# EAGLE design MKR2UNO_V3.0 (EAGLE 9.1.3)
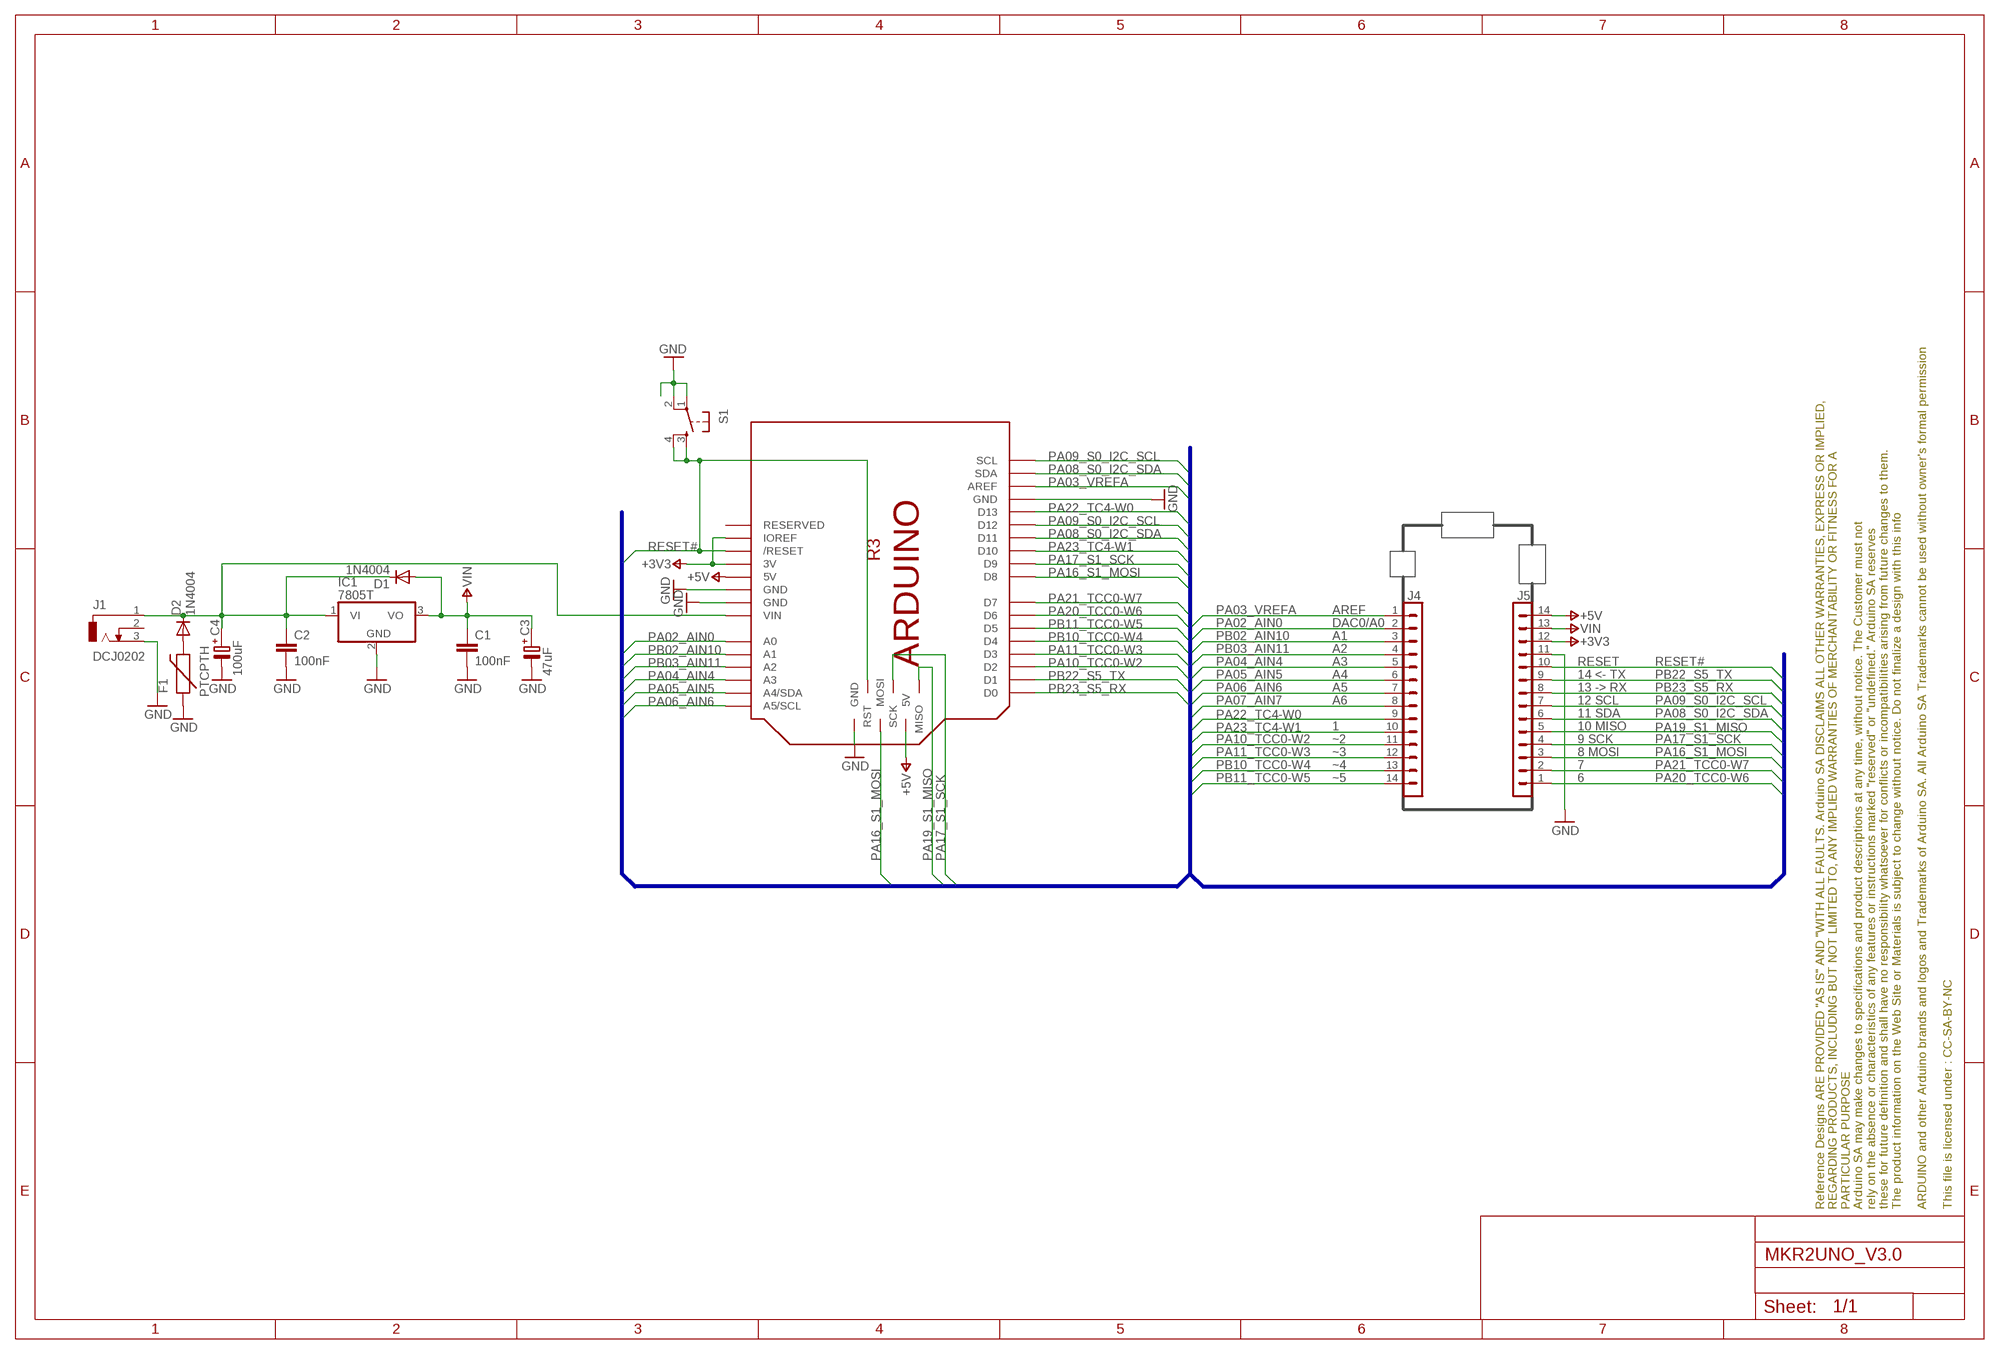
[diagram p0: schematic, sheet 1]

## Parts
C1  100nF  C-EU025-024X044  [C025-024X044]
C2  100nF  C-EU025-024X044  [C025-024X044]
C3  47uF  C-PA-6,3X10  [EA6,3-10]
C4  100uF  C-PA-6,3X10  [EA6,3-10]
D1  1N4004  [DO41-10]
D2  1N4004  [DO41-10]
F1  PTCPTH  [PTC]
FRAME1  DNP  A3-FRAME-STANDARD  [FRAME]
IC1  7805T  [TO220H]
J1  DCJ0202  [DCJ0202]
J4  DNP  STRIP-14STD  [1X14]
J5  DNP  STRIP-14STD  [1X14]
M1  ARDUINO_R3_ICSP  [ARDUINOR3_ICSP]
S1  TAC_SWITCHPTH  [TACTILE-PTH]

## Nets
+3V3: J5.12 M1.3V M1.IOREF
+5V: J5.14 M1.5V M1.5V_ICSP(5V)
GND: C1.2 C2.2 C3.- C4.- F1.P$1 IC1.2(GND) J1.3 J5.11 M1.GND M1.GND@1(GND) M1.GND@2(GND) M1.GND@3(GND) S1.1 S1.2
N$1: C2.1 C4.+ D1.C D2.C IC1.1(VI) J1.1 M1.VIN
N$2: D2.A F1.P$2
PA02_AIN0: J4.2 M1.A0
PA03_VREFA: J4.1 M1.AREF
PA04_AIN4: J4.5 M1.A3
PA05_AIN5: J4.6 M1.A4(A4/SDA)
PA06_AIN6: J4.7 M1.A5(A5/SCL)
PA07_AIN7: J4.8
PA08_S0_I2C_SDA: J5.6 M1.D11 M1.SDA
PA09_S0_I2C_SCL: J5.7 M1.D12 M1.SCL
PA10_TCC0-W2: J4.11 M1.D2
PA11_TCC0-W3: J4.12 M1.D3
PA16_S1_MOSI: J5.3 M1.D8 M1.MOSI
PA17_S1_SCK: J5.4 M1.D9 M1.SCK
PA19_S1_MISO: J5.5 M1.MISO
PA20_TCC0-W6: J5.1 M1.D6
PA21_TCC0-W7: J5.2 M1.D7
PA22_TC4-W0: J4.9 M1.D13
PA23_TC4-W1: J4.10 M1.D10
PB02_AIN10: J4.3 M1.A1
PB03_AIN11: J4.4 M1.A2
PB10_TCC0-W4: J4.13 M1.D4
PB11_TCC0-W5: J4.14 M1.D5
PB22_S5_TX: J5.9 M1.D1
PB23_S5_RX: J5.8 M1.D0
RESET#: J5.10 M1.RESET(/RESET) M1.RESET_ICSP(RST) S1.3 S1.4
VIN: C1.1 C3.+ D1.A IC1.3(VO) J5.13
Unconnected: J1.2 M1.RESERVED

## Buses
PA03_VREFA,PA02_AIN0,PB02_AIN10,PB03_AIN11PA04_AIN4,PA05_AIN5,PA06_AIN6,PA07_AIN7,PA22_TC4-W0,PA23_TC4-W1,PA10_TCC0-W2,PA11_TCC0-W3,PB10_TCC0-W4,PB11_TCC0-W5,PA20_TCC0-W6,PA21_TCC0-W7,PA16_S1_MOSI,PA17_S1_SCK,PA19_S1_MISO,PA08_S0_I2C_SDA,PA09_S0_I2C_SCL,PB23_S5_RX,PB22_S5_TX,RESET#

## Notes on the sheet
- AREF
- DAC0/A0
- A1
- A2
- A3 | RESET
- A4 | 14 <- TX
- A5 | 13 -> RX
- A6 | 12 SCL
- 11 SDA
- 1 | 10 MISO
- ~2 | 9 SCK
- ~3 | 8 MOSI
- ~4 | 7
- ~5 | 6

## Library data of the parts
C1 C2 = rcl:C-EU: CAPACITOR, European symbol
C3 C4 = cap-pan40:C-PA: POLARIZED AXIAL ELECTROLYTIC
D1 D2 = diode:1N4004: DIODE
F1 = SparkFun:PTC: Resettable Fuse PTC
FRAME1 = Arduino-utility:A3-FRAME: Schematic frame; CODE-ARDUINO: DNP; DATASHEET: DNP; DISTRIBUTOR-LINK: DNP; DISTRIBUTOR-PN: DNP; MANUFACTURER: DNP; MANUFACTURER-PN: DNP
IC1 = linear:78*: Positive VOLTAGE REGULATOR Source: http://cache.national.com/ds/LM/LM78L05.pdf http://www.fairchildsemi.com/ds/LM/LM7805.pdf
J1 = con-jack:DCJ0202: DC POWER JACK Source: DCJ0202.pdf
J4 J5 = Arduino-connectors:STRIP-14
M1 = Arduino-BoardFootprints:ARDUINO_R3_ICSP
S1 = SparkFun:TAC_SWITCH: Momentary Switch Button commonly used for reset or general input. Spark Fun Electronics SKU : COM-00097

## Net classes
0 default: width 0.25 mm, drill 0.25 mm

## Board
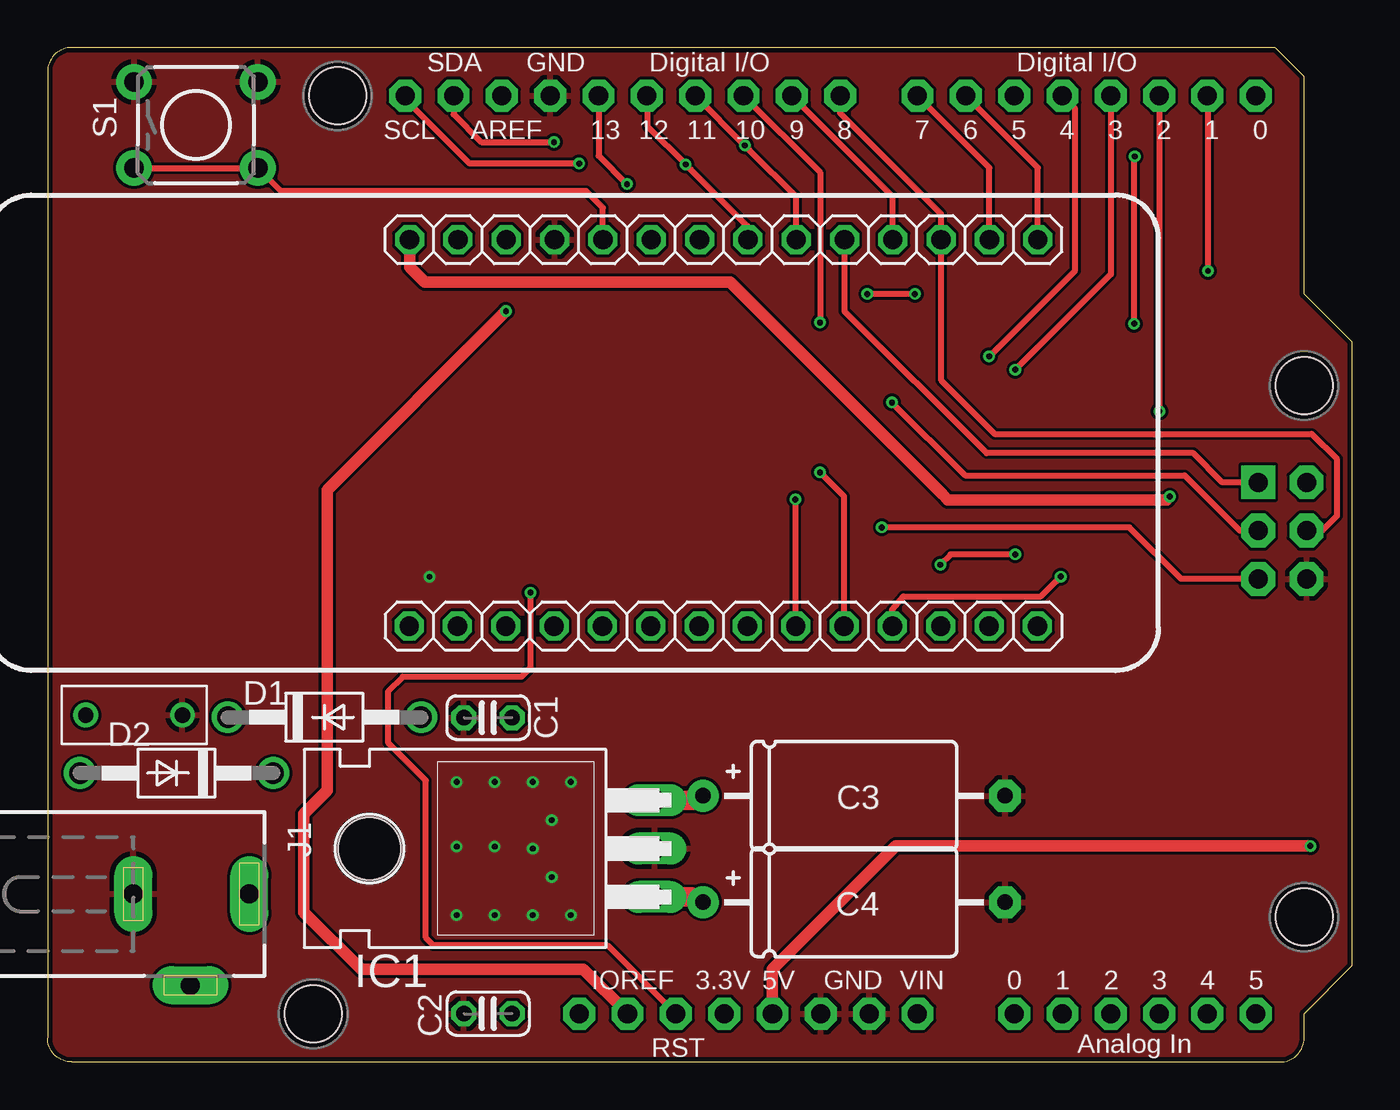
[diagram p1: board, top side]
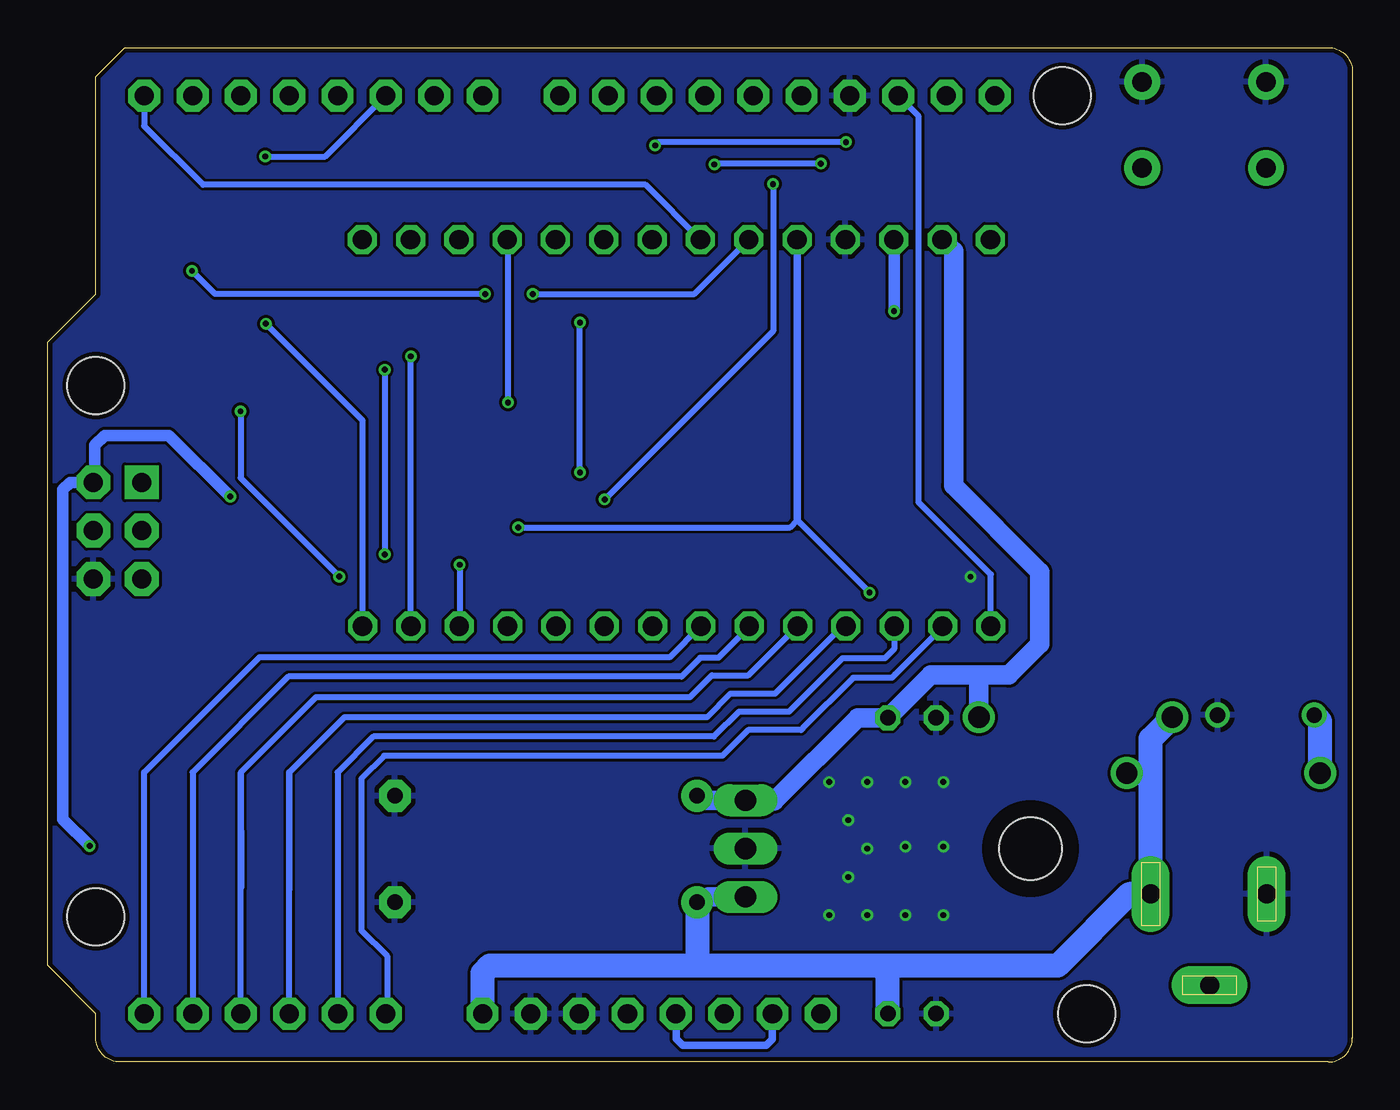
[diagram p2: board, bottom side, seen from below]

Size 68.58 x 53.34 mm. Coordinates in mm from the lower left corner, seen from the top.
Copper layers (1*16): Top 0.035mm / dielectric 1.5mm / Bottom 0.035mm
Design rules "SeeedStudio_2layers *": minimum track width 6mil, minimum drill 12mil, track to track 6mil, track to pad 6mil, pad to pad 6mil, via to via 6mil, smd to smd 0mil, copper to edge 10mil, drill to drill 10mil, minimum pad ring 10mil, minimum via ring 6mil, stop-mask expansion 2mil, vias tented up to drill 100mil, thermal gap 10mil

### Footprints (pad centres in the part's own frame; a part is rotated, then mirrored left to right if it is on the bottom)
C025-024X044 = drill 0.813 octagon: 1 -1.27,0; 2 1.27,0
EA6,3-10 = drill 0.813 pad 1.676: + -8.255,0 | drill 0.813 pad 1.676 octagon: - 7.62,0
DO41-10 = drill 1.118: A 5.08,0; C -5.08,0
PTC = drill 0.8: P$1 -2.54,0; P$2 2.54,0
TO220H = drill 1.118 long: 1 -2.54,-10.16; 2 0,-10.16; 3 2.54,-10.16 | hole 3.302: 0,4.826
DCJ0202 = drill 1 pad 2 long: 1 0,3.1; 2 4.8,0; 3 0,-3
1X14 = drill 1.016 octagon: 1 -16.51,0; 2 -13.97,0; 3 -11.43,0; 4 -8.89,0; 5 -6.35,0; 6 -3.81,0; 7 -1.27,0; 8 1.27,0; 9 3.81,0; 10 6.35,0; 11 8.89,0; 12 11.43,0; 13 13.97,0; 14 16.51,0
ARDUINOR3_ICSP = drill 1 pad 1.676 octagon: 3V 35.56,2.54; 5V 38.1,2.54; A0 50.8,2.54; A1 53.34,2.54; A2 55.88,2.54; A3 58.42,2.54; A4 60.96,2.54; A5 63.5,2.54; AREF 23.876,50.8; D0 63.5,50.8; D1 60.96,50.8; D2 58.42,50.8; D3 55.88,50.8; D4 53.34,50.8; D5 50.8,50.8; D6 48.26,50.8; D7 45.72,50.8; D8 41.656,50.8; D9 39.116,50.8; D10 36.576,50.8; D11 34.036,50.8; D12 31.496,50.8; D13 28.956,50.8; GND 26.416,50.8; GND@1 43.18,2.54; GND@2 40.64,2.54; IOREF 30.48,2.54; RESERVED 27.94,2.54; RESET 33.02,2.54; SCL 18.796,50.8; SDA 21.336,50.8; VIN 45.72,2.54 | drill 1 pad 1.778 octagon: 5V_ICSP 66.167,30.48; GND@3 66.167,25.4; MOSI 66.167,27.94; RESET_ICSP 63.627,25.4; SCK 63.627,27.94 | drill 1 pad 1.778 square: MISO 63.627,30.48 | hole 3: 15.24,50.8; 13.97,2.54; 66.04,7.62; 66.04,35.56
TACTILE-PTH = drill 1.016 pad 1.88: 1 -3.251,2.261; 2 3.251,2.261; 3 -3.251,-2.261; 4 3.251,-2.261

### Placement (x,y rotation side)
C1  23.15,18.1 180 top
C2  23.15,2.54 180 top
C3  42.7,14 0 top
C4  42.7,8.4 0 top
D1  14.55,18.13 0 top
D2  6.78,15.19 180 top
F1  4.55,18.24 180 top
FRAME1  not placed on the board
IC1  21.74,11.22 90 top
J1  7.51,8.83 270 top
J4  35.51,22.92 0 top
J5  35.53,43.24 180 top
M1  0,0 0 top
S1  7.8,49.27 0 top

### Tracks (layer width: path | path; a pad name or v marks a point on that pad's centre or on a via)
+3V3  (via drill 0.3 pad 0.61)
  Top 0.61: M1.IOREF 28.16,4.87 16.48,4.87 13.47,7.88 13.47,13.05 14.69,14.27 14.69,30.08 v24.09,39.48 24.07,39.5
  Bottom 0.406: M1.IOREF 30.48,1.19 30.8,0.87 35.19,0.87 35.54,1.22 35.54,2.52 M1.3V
  Bottom 0.61: v24.09,39.48 24.09,43.23 J5.12
+5V  (via drill 0.3, 0.3 pad 0.61)
  Top 0.61: v58.98,29.73 58.81,29.56 47.31,29.56 47.04,29.83 47.04,29.84 35.87,41.01 19.82,41.01 19.02,41.8 J5.14 | v66.37,11.36 46.92,11.36 46.91,11.37 44.59,11.37 38.1,4.88 M1.5V
  Bottom 0.61: v58.98,29.73 62.2,32.95 65.58,32.95 66.1,32.43 66.1,30.55 M1.5V_ICSP 67.4,30.48 67.77,30.11 67.77,12.76 v66.37,11.36
GND  (via drill 0.3)
  other vias: 27.5,7.72 25.5,7.72 23.5,7.72 21.5,7.72 27.5,14.72 26.5,12.72 26.5,9.72 25.5,11.22 23.5,11.32 21.5,11.32 25.5,14.72 23.5,14.72 21.5,14.72 20.07,25.51
  pour Bottom: 0,55 70,55 70,0 0,0
  pour Top: 0,55 70,55 70,0 0,0
N$1
  Top 1.016: IC1.1 33.84,8.68 C4.+
  Bottom 0.406: 16.69,5.07 16.74,5.07 16.74,5.4
  Bottom 1.016: 34.12,5.13 34.05,5.07 | C4.+ 33.84,8.68 31.82,8.68
  Bottom 1.27: M1.VIN 45.72,4.67 45.32,5.07 34.05,5.07 24.85,5.07 | 24.85,5.07 16.69,5.07 16.68,5.06 15.5,5.06 11.73,8.83 J1.1 10.61,14.94 | C2.1 24.42,4.64 24.85,5.07 | 10.61,14.94 10.61,16.99 D1.C | C4.+ 34.45,5.46 34.12,5.13 | D2.C 10.86,15.19 10.61,14.94
N$2
  Bottom 1.27: D2.A 1.7,17.93 F1.P$2
PA02_AIN0
  Bottom 0.305: J4.2 21.55,22.88 24.03,20.39 24.03,20.38 24.21,20.2 26.24,20.2 28.88,17.56 28.88,17.55 28.98,17.45 31.76,17.45 33.11,16.1 50.89,16.1 52.09,14.9 52.09,6.92 50.74,5.57 50.74,2.6 M1.A0
PA03_VREFA
  Bottom 0.305: M1.AREF 22.8,49.72 22.8,29.43 19,25.64 J4.1
PA04_AIN4
  Bottom 0.305: 58.49,2.61 M1.A3 58.42,15.23 | J4.5 31.75,20.33 33.66,20.33 34.82,19.17 54.48,19.17 58.42,15.23 | 58.42,15.23 58.41,9.15
PA05_AIN5
  Bottom 0.305: 31.68,22.89 J4.6 31.7,22.86 33.32,21.25 34.28,21.25 35.26,20.27 55.92,20.27 60.96,15.23 M1.A4
PA06_AIN6
  Bottom 0.305: 34.23,22.91 J4.7 35.88,21.28 57.45,21.28 63.5,15.23 M1.A5
PA08_S0_I2C_SDA  (via drill 0.3, 0.3 pad 0.6)
  Top 0.305: J5.6 39.34,45.49 36.89,47.95 v36.65,48.19 M1.D11 | M1.SDA 21.34,49.83 22.8,48.37 v26.62,48.37
  Bottom 0.305: 39.27,43.32 J5.6 | v26.62,48.37 36.47,48.37 v36.65,48.19
PA09_S0_I2C_SCL  (via drill 0.3, 0.3 pad 0.6)
  Top 0.305: J5.7 36.79,43.23 36.78,43.23 36.78,43.95 33.81,46.92 v33.53,47.2 31.55,49.18 31.55,50.75 M1.D12 | M1.SCL 18.8,50.62 22.17,47.25 v27.93,47.25 v27.94,47.24
  Bottom 0.305: v27.94,47.24 33.49,47.24 v33.53,47.2
PA10_TCC0-W2  (via drill 0.3 pad 0.6)
  Top 0.305: M1.D2 58.43,47.9 v58.43,34.22 v58.44,34.21 | J4.11 44.38,22.95 44.38,23.78 44.98,24.48 52.21,24.48 53.02,25.29 | 53.02,25.29 53.02,25.28 | 53.02,25.29 v53.25,25.52
  Bottom 0.305: v58.44,34.21 58.44,30.71 v53.25,25.52
PA11_TCC0-W3  (via drill 0.3)
  Top 0.305: v50.86,26.69 47.46,26.69 v46.92,26.15 | M1.D3 55.88,41.42 v50.86,36.4
  Bottom 0.305: v50.86,36.4 v50.86,26.69 | v46.92,26.15 46.92,22.95 J4.12
PA16_S1_MOSI
  Top 0.305: 46.98,43.22 46.98,35.83 49.78,33.03 66.44,33.03 67.78,31.69 67.78,28.73 66.99,27.94 M1.MOSI | M1.D8 41.66,49.89 46.97,44.59 J5.3
  Top 0.406: 46.98,43.22 J5.3
PA17_S1_SCK  (via drill 0.3)
  Top 0.305: 44.39,43.2 J5.4 44.42,45.49 M1.D9 | M1.SCK 62.66,27.94 59.76,30.84 48.22,30.84 v44.38,34.68
  Bottom 0.305: v44.38,34.68 44.38,43.2
  Bottom 0.406: 44.38,43.2 J5.4
PA19_S1_MISO
  Top 0.305: M1.MISO 61.75,30.48 60.22,32.01 49.35,32.01 41.88,39.48 J5.5
PA20_TCC0-W6
  Top 0.305: J5.1 52.05,47.02 M1.D6
PA21_TCC0-W7
  Top 0.305: J5.2 49.51,47.02 M1.D7
PA22_TC4-W0  (via drill 0.3 pad 0.6)
  Top 0.305: M1.D13 28.96,47.65 v30.45,46.16 | v39.3,29.58 39.3,22.95 J4.9
  Bottom 0.305: v30.45,46.16 30.45,38.43 v39.3,29.58
PA23_TC4-W1  (via drill 0.3 pad 0.6)
  Top 0.305: M1.D10 40.6,46.78 v40.6,38.88 | J4.10 41.87,29.73 v40.6,31
  Bottom 0.305: v40.6,31 v40.6,38.88
PB02_AIN10
  Bottom 0.305: J4.3 24.09,21.7 24.57,21.22 26.81,21.22 29.6,18.43 32.24,18.43 33.56,17.11 51.46,17.11 53.34,15.23 M1.A1
PB03_AIN11
  Bottom 0.305: 55.95,2.61 M1.A2 55.88,15.23 | J4.4 26.79,22.92 30.34,19.37 32.69,19.37 33.93,18.13 52.98,18.13 55.88,15.23 | 55.88,15.23 55.89,9.02
PB10_TCC0-W4  (via drill 0.3)
  Top 0.305: v49.48,37.1 54,41.62 54,50.14 M1.D4
  Bottom 0.305: J4.13 v49.48,37.1
PB11_TCC0-W5  (via drill 0.3 pad 0.6)
  Top 0.305: v57.11,38.82 57.11,47.58 v57.14,47.61
  Bottom 0.305: J4.14 52.02,33.73 v57.11,38.82 | v57.14,47.61 53.99,47.61 M1.D5
PB22_S5_TX  (via drill 0.3)
  Top 0.305: v45.58,40.38 v43.08,40.38 | v60.99,41.6 60.99,50.77 M1.D1
  Bottom 0.305: v43.08,40.38 34.59,40.38 J5.9 | 45.58,40.28 v45.58,40.38 59.77,40.38 v60.99,41.6
PB23_S5_RX
  Bottom 0.305: M1.D0 63.5,49.21 60.41,46.12 37.15,46.12 J5.8
RESET#  (via drill 0.3, 0.3 pad 0.6)
  Top 0.305: M1.RESET 29.43,6.13 20.28,6.13 19.88,6.53 19.88,14.8 17.91,16.77 17.91,19.5 18.66,20.25 24.9,20.25 25.38,20.73 v25.38,24.68 | S1.3 S1.4 12.27,45.79 28.31,45.79 29.18,44.91 J5.10 | M1.RESET_ICSP 59.57,25.4 56.86,28.11 v43.84,28.11
  Bottom 0.305: v25.38,24.68 29.18,28.48 29.56,28.11 v43.84,28.11
  Bottom 0.406: J5.10 29.18,28.48
VIN
  Top 1.016: IC1.3 33.88,13.76 C3.+
  Bottom 1.016: J5.13 20.96,42.63 20.96,30.3 16.43,25.77 16.43,21.97 18.05,20.35 19.64,20.35 | C3.+ 33.88,13.76 31.76,13.76 31.74,13.74 | IC1.3 31.04,13.72 30.38,13.72 26,18.1 C1.1 22.17,20.35 19.64,20.35 | 19.64,20.35 19.71,20.28 19.63,20.2 D1.A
